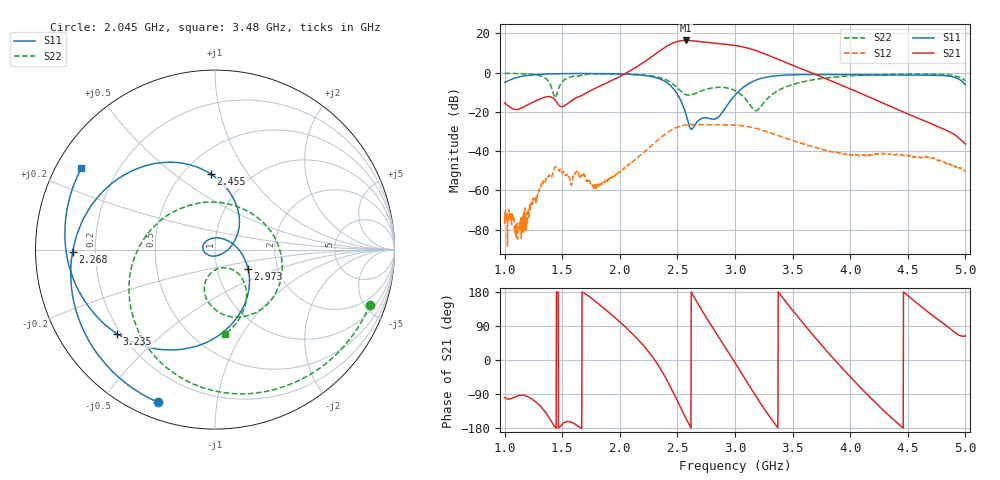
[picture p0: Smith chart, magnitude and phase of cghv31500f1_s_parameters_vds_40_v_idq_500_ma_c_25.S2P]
!Keysight Technologies,E5071C,MY46632031,B.14.03
!Date: Fri Jul 09 16:07:18 2021
!Data & Calibration Information:
!Freq	S11:SOLT2(ON)	S21:SOLT2(ON)	S12:SOLT2(ON)	S22:SOLT2(ON)
!PortZ  Port1:50+j0  Port2:50+j0
!Above PortZ is port z conversion or system Z0 setting when saving the data.
!When reading, reference impedance value at option line is always used.
# Hz S dB R 50
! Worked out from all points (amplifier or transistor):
!   1601 points, 1 GHz to 5 GHz, reference 50 ohm
!   highest |S21| = 16.3 dB at 2.575 GHz (marker M1)
!   |S21| within 3 dB of that: 2.406 GHz to 3.045 GHz (638.9 MHz wide, 23.4 % of centre)
!   unconditionally stable (mu >= 1): start of sweep to end of sweep
!   at 1.665 GHz: K = 25.49, MAG = 3.2 dB, |S12| = -52.5 dB
!   at 3 GHz: K = 1.85, MAG = 14.9 dB, |S12| = -26.7 dB
!   at 5 GHz: K = 5142.32, MAG = -33.3 dB, |S12| = -50.2 dB
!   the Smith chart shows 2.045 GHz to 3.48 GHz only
!   S11 on the Smith chart (normalised r, x): 2.045 GHz: 0.07, -0.69; 2.268 GHz: 0.12, -0.01; 2.455 GHz: 0.68, +0.69; 2.973 GHz: 1.41, -0.31; 3.235 GHz: 0.18, -0.36; 3.48 GHz: 0.07, +0.28
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1e9  -5.01 154.1  -15.38 -99.2  -73.19 150.0  -0.40 122.2
1.315e9  -0.90 75.4  -13.27 -123.4  -58.05 -136.8  -1.75 61.2
1.6675e9  -0.50 -15.3  -11.74 -179.5  -52.45 -168.1  -1.47 54.7
2.045e9  -0.84 -110.5  -0.58 88.1  -48.61 6.9  -0.76 -19.5
2.2675e9  -2.01 -179.1  7.70 14.8  -37.65 -67.9  -1.60 -73.7
2.335e9  -2.99 153.9  10.54 -14.6  -34.24 -98.1  -2.32 -97.0
2.4e9  -4.80 123.0  13.13 -48.0  -31.18 -132.0  -3.63 -125.3
2.455e9  -7.53 92.9  14.89 -80.3  -29.06 -164.3  -5.61 -156.0
2.5125e9  -12.30 57.2  15.99 -116.2  -27.56 159.7  -8.50 163.4
2.575e9  -21.34 8.1  16.34 -154.4  -26.75 121.6  -11.27 106.6
2.655e9  -26.51 -139.5  16.05 160.6  -26.52 76.2  -10.69 39.9
2.765e9  -23.27 142.6  15.30 105.3  -26.60 21.3  -8.34 -12.1
2.855e9  -22.76 58.3  14.73 62.5  -26.64 -21.1  -7.51 -43.2
2.9725e9  -13.45 -30.0  14.00 6.5  -26.66 -76.7  -8.49 -79.5
3e9  -11.51 -43.7  13.77 -7.0  -26.73 -90.0  -9.22 -87.4
3.115e9  -5.82 -93.8  12.38 -63.6  -27.64 -146.1  -15.31 -106.1
3.235e9  -2.85 -139.3  10.02 -120.4  -29.40 157.3  -16.47 -48.6
3.335e9  -1.79 -171.6  7.66 -163.8  -31.26 113.7  -10.61 -53.5
3.48e9  -1.20 148.7  4.19 138.7  -34.23 55.9  -6.49 -83.3
3.6675e9  -1.03 103.9  -0.22 69.3  -37.62 -11.5  -3.79 -129.4
4.335e9  -1.29 -65.3  -16.89 -145.9  -41.79 176.9  -0.94 62.3
5e9  -6.24 120.2  -36.48 63.7  -50.21 36.8  -4.25 -50.1
